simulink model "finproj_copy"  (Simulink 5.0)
settings: Solver=ode45  StartTime=0.0  StopTime=100.0  RelTol=1e-3
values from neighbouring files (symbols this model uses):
  denp = (abs(denp)>1e-8).*denp    [segway.m]
  nump = [nump 0]/numv(2)    [segway.m]

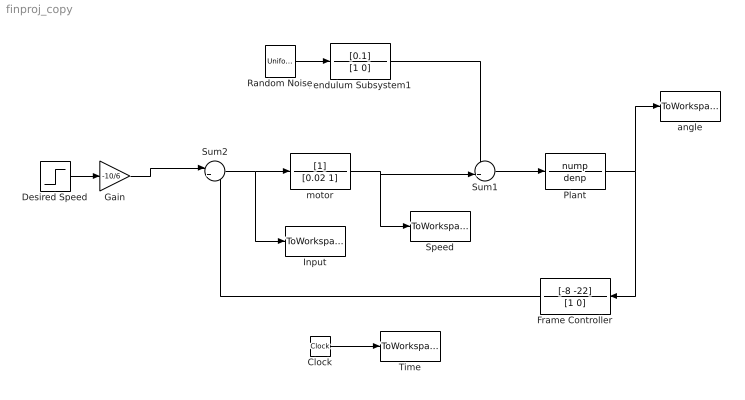
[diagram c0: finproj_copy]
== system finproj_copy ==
  Clock : Clock
  Desired Speed : Step  Time=0  After=2  SampleTime=0
  Frame Controller : TransferFcn  Orientation=left  Numerator=[-8 -22]  Denominator=[1 0]
  Gain : Gain  Gain=-10/6
  Input : ToWorkspace  VariableName=u  SampleTime=-1  SaveFormat=Array
  Pendulum Subsystem1 : TransferFcn  Numerator=[0.1]  Denominator=[1 0]
  Plant : TransferFcn  Numerator=nump  Denominator=denp
  Random Noise : UniformRandomNumber  SampleTime=0
  Speed : ToWorkspace  VariableName=v  SampleTime=-1  SaveFormat=Array
  Sum1 : Sum  Inputs=++|
  Sum2 : Sum  Inputs=|+-
  Time : ToWorkspace  VariableName=t  SampleTime=-1  SaveFormat=Array
  angle : ToWorkspace  VariableName=th  SampleTime=-1  SaveFormat=Array
  motor : TransferFcn  Denominator=[0.02 1]
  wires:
  Plant/1 -> Frame Controller/1, angle/1
  Clock/1 -> Time/1
  Sum2/1 -> motor/1, Input/1
  Gain/1 -> Sum2/1
  Frame Controller/1 -> Sum2/2
  Random Noise/1 -> Pendulum Subsystem1/1
  Pendulum Subsystem1/1 -> Sum1/1
  Sum1/1 -> Plant/1
  motor/1 -> Sum1/2, Speed/1
  Desired Speed/1 -> Gain/1
